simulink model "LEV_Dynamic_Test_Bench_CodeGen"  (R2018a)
settings: Solver=VariableStepAuto  StartTime=0  StopTime=37  RelTol=1e-3
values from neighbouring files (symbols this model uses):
  Anglog_Input_Max = 10    [Panda_BEVintage_VPE_S_Data_CodeGen_Model.m]    (also in ParameterInitializationFileFinal.m = 3; Panda_BEVintage_VPE_S_Data_Enhanced_Model.m)
  Anglog_Input_Min = -10    [Panda_BEVintage_VPE_S_Data_CodeGen_Model.m]    (also in ParameterInitializationFileFinal.m = 0; Panda_BEVintage_VPE_S_Data_Enhanced_Model.m)
  Anglog_Output_Max = 10    [Panda_BEVintage_VPE_S_Data_CodeGen_Model.m]    (also in Panda_BEVintage_VPE_S_Data_Enhanced_Model.m)
  Anglog_Output_Min = -10    [Panda_BEVintage_VPE_S_Data_CodeGen_Model.m]    (also in Panda_BEVintage_VPE_S_Data_Enhanced_Model.m)
  Bits = 16    [Panda_BEVintage_VPE_S_Data_CodeGen_Model.m]    (also in ParameterInitializationFileFinal.m = 12; Panda_BEVintage_VPE_S_Data_Enhanced_Model.m)
  c_1 = 0    [Panda_BEVintage_VPE_S_Data_CodeGen_Model.m]    (also in Panda_BEVintage_VPE_S_Data_Enhanced_Model.m)
  Full_BTrq_Range = Max_BTrq-Min_BTrq    (= 132)    [Panda_BEVintage_VPE_S_Data_CodeGen_Model.m]    (also in Panda_BEVintage_VPE_S_Data_Enhanced_Model.m)
  Full_Scale_Reading = Anglog_Input_Max-Anglog_Input_Min    (= 20)    [Panda_BEVintage_VPE_S_Data_CodeGen_Model.m]    (also in ParameterInitializationFileFinal.m = 3; Panda_BEVintage_VPE_S_Data_Enhanced_Model.m)
  Full_Speed_Range = Max_Speed-Min_Speed    (= 2513.27412287)    [Panda_BEVintage_VPE_S_Data_CodeGen_Model.m]    (also in Panda_BEVintage_VPE_S_Data_Enhanced_Model.m)
  g = 9.81    [Panda_BEVintage_VPE_S_Data_CodeGen_Model.m]    (also in Panda_BEVintage_VPE_S_Data_Enhanced_Model.m)
  m_e = 1.0359e+03    (= 1035.9)    [Panda_BEVintage_VPE_S_Data_CodeGen_Model.m]    (also in Panda_BEVintage_VPE_S_Data_Enhanced_Model.m)
  Max_BTrq = T_m_max    (= 66)    [Panda_BEVintage_VPE_S_Data_CodeGen_Model.m]    (also in Panda_BEVintage_VPE_S_Data_Enhanced_Model.m)
  Max_Speed = 400*pi    (= 1256.63706144)    [Panda_BEVintage_VPE_S_Data_CodeGen_Model.m]    (also in Panda_BEVintage_VPE_S_Data_Enhanced_Model.m)
  MaxInputBTrq = 5    [Panda_BEVintage_VPE_S_Data_CodeGen_Model.m]    (also in Panda_BEVintage_VPE_S_Data_Enhanced_Model.m)
  MaxOutputSpeedSensor = 5    [Panda_BEVintage_VPE_S_Data_CodeGen_Model.m]    (also in Panda_BEVintage_VPE_S_Data_Enhanced_Model.m)
  Min_BTrq = -T_m_max    (= -66)    [Panda_BEVintage_VPE_S_Data_CodeGen_Model.m]    (also in Panda_BEVintage_VPE_S_Data_Enhanced_Model.m)
  Min_Speed = -400*pi    (= -1256.63706144)    [Panda_BEVintage_VPE_S_Data_CodeGen_Model.m]    (also in Panda_BEVintage_VPE_S_Data_Enhanced_Model.m)
  MinInputBTrq = -5    [Panda_BEVintage_VPE_S_Data_CodeGen_Model.m]    (also in Panda_BEVintage_VPE_S_Data_Enhanced_Model.m)
  MinOutputSpeedSensor = -5    [Panda_BEVintage_VPE_S_Data_CodeGen_Model.m]    (also in Panda_BEVintage_VPE_S_Data_Enhanced_Model.m)
  r_e = 0.27    [Panda_BEVintage_VPE_S_Data_CodeGen_Model.m]    (also in Panda_BEVintage_VPE_S_Data_Enhanced_Model.m)
  Sampling_Time = 0.0001    [Panda_BEVintage_VPE_S_Data_CodeGen_Model.m]    (also in ParameterInitializationFileFinal.m = 0.01; Panda_BEVintage_VPE_S_Data_Enhanced_Model.m)
  T_m_max = 66    [Panda_BEVintage_VPE_S_Data_CodeGen_Model.m]    (also in Panda_BEVintage_VPE_S_Data_Enhanced_Model.m)
  T_r = 8.67    [Panda_BEVintage_VPE_S_Data_CodeGen_Model.m]    (also in Panda_BEVintage_VPE_S_Data_Enhanced_Model.m)
  ZOH_Time = 0.0001    [Panda_BEVintage_VPE_S_Data_CodeGen_Model.m]    (also in Panda_BEVintage_VPE_S_Data_Enhanced_Model.m)
undefined symbols (not defined in the file or in its folder): DiscIntNeverNeededParam, m, s, seconds
libraries: autolibmappedmotor x2, simulink x2, autolibshared x2, autolibsharedcoupling x1

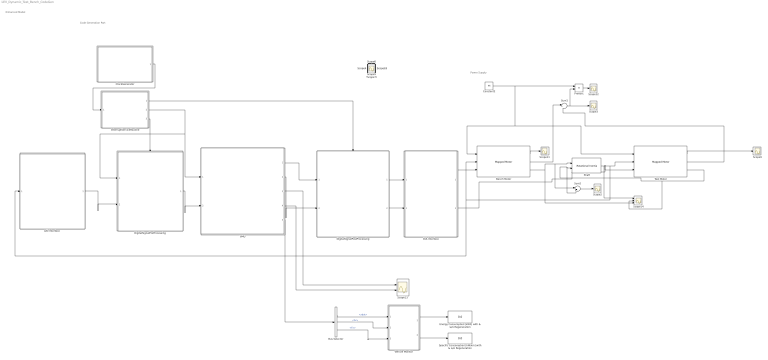
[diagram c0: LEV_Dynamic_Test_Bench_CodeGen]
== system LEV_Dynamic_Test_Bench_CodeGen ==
  note: Enhanced Model
  note: Code Generation Part
  note: Power Supply
  "A/D Interface " : Subsystem
  Bench Motor : autolibmappedmotor/Mapped Motor  port_config=Speed  param_by=Maximum torque and power  w_t=[ 0 375 750 800 ]  T_t=[0.09 0.08 0.07 0]  torque_max=T_m_max  power_max=P_m_max  Tc=tau_m  param_loss=Single efficiency measurement  eff=eta_n  w_eff=w_n  T_eff=T_m_n  Piron=Pl_iron  Pbase=Pl_eln  w_eff_bp=[-8000 -4000 0 4000 8000]  T_eff_bp=[0 0.03 0.06 0.09]  losses_table=[1 2;3 4]  efficiency_table=[95 95 95 95; 95 95 95 95; 95 95 95 95; 95 95 95 95; 95 95 95 95]  J=5e-6  b=1e-5  omega_o=0  T_t_extended=[0 0.07 0.08 0.09 0.08 0.07 0]  w_t_extended=[-800 -750 -375 0 375 750 800]  KLossIron=0  KLossCopper=0.68708  x_w_eff_vec=[-400 0 400]  x_T_eff_vec=[-20 0 20]  x_losses_mat=[4 3 4;2 1 2;4 3 4]  aMode=aMode
  Bus Selector : BusSelector  OutputSignals=BdyFrm.Cg.Vel.xdot,BdyFrm.Forces.Ext.Fx,BdyFrm.Forces.Drag.Fx
  ClockGenerator : Subsystem
  Constant2 : Constant  Value=96
  D/A Interface : Subsystem
  DigitalSignalPostProcessing : Subsystem
  DigitalSignalPreProcessing : Subsystem
  Energy Consumption [kWh] with & w/o Regeneration : Display
  InterruptServiceRoutine : Subsystem
  Product : Product
  Scope{,1..12,18} (14 alike) : Scope
  Scope13 : Scope  NumInputPorts=2
  Scope14 : Scope  NumInputPorts=3
  Shaft : autolibsharedcoupling/Rotational Inertia  port_config=Simulink  J=.01  b=.001  omega_o=0  externJ=off  blkID=0  aMode=1
  Specific Consumption [kW/km] with & w/o Regeneration : Display
  Sum1 : Sum  Inputs=|++
  Sum2 : Sum  Inputs=|++
  Test Motor : autolibmappedmotor/Mapped Motor  port_config=Speed  param_by=Maximum torque and power  w_t=[ 0 375 750 800 ]  T_t=[0.09 0.08 0.07 0]  torque_max=T_m_max  power_max=P_m_max  Tc=tau_m  param_loss=Single efficiency measurement  eff=eta_n  w_eff=w_n  T_eff=T_m_n  Piron=Pl_iron  Pbase=Pl_eln  w_eff_bp=[-8000 -4000 0 4000 8000]  T_eff_bp=[0 0.03 0.06 0.09]  losses_table=[1 2;3 4]  efficiency_table=[95 95 95 95; 95 95 95 95; 95 95 95 95; 95 95 95 95; 95 95 95 95]  J=5e-6  b=1e-5  omega_o=0  T_t_extended=[0 0.07 0.08 0.09 0.08 0.07 0]  w_t_extended=[-800 -750 -375 0 375 750 800]  KLossIron=0  KLossCopper=0.68708  x_w_eff_vec=[-400 0 400]  x_T_eff_vec=[-20 0 20]  x_losses_mat=[4 3 4;2 1 2;4 3 4]  aMode=aMode
  VMU : Subsystem
  Vehicle Monitor : Subsystem
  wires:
  Test Motor/3 -> Scope14/2, Shaft/2, Sum2/2
  Bench Motor/3 -> Scope14/3, Sum2/1, Shaft/1
  Constant2/1 -> Bench Motor/1, Test Motor/1, Product/1
  Shaft/1 -> Scope14/1, "A/D Interface "/1(ShaftSpeed), Bench Motor/2, Test Motor/2
  Test Motor/2 -> Sum1/2
  Sum1/1 -> Product/2, Scope3/1
  Bench Motor/2 -> Sum1/1
  Sum2/1 -> Scope2/1
  Bench Motor/1 -> Scope11/1
  Test Motor/1 -> Scope9/1
  Product/1 -> Scope12/1
  Bus Selector/1 -> Vehicle Monitor/1(In1)  "<xdot>"
  Bus Selector/3 -> Vehicle Monitor/3(In3)  "<Fx>"
  Bus Selector/2 -> Vehicle Monitor/2(In2)  "<Fx>"
  Vehicle Monitor/1(Out1) -> Energy Consumption [kWh] with & w/o Regeneration/1
  Vehicle Monitor/2(Out2) -> Specific Consumption [kW/km] with & w/o Regeneration/1
  D/A Interface/1("BenchTrqCMD ") -> Bench Motor/3
  D/A Interface/2("MotorTrqCMD ") -> Test Motor/3
  VMU/3(Speed [m/s]) -> Scope13/1
  VMU/4(ForceTot) -> Scope13/2
  VMU/5(VehicleBodyInfo) -> Bus Selector/1
  "A/D Interface "/1(ShaftSpeedDigitalSignal) -> DigitalSignalPreProcessing/2(ShaftSpeedDigitalSignal)
  DigitalSignalPreProcessing/1("AverageShaftSpeedDigitalSignal ") -> VMU/2("AverageShaftSpeedDigitalSignal ")
  ClockGenerator/1(ClkSignal) -> InterruptServiceRoutine/1(ClkSignal)
  DigitalSignalPostProcessing/1(BenchTrqCMD16Bits) -> D/A Interface/1(DigitalBenchTrqCMD)
  DigitalSignalPostProcessing/2(MotorTrqCMD16Bits) -> D/A Interface/2(DigitalMotorTrqCMD)
  VMU/2(MotorTrqCMD) -> DigitalSignalPostProcessing/2(MotorTrqCMD)
  VMU/1(BenchTrqCMD) -> DigitalSignalPostProcessing/1(BenchTrqCMD)
  InterruptServiceRoutine/2(CoreTrigger) -> VMU/1(ClkVMU), DigitalSignalPreProcessing/1(PeriodicAvgExtraction)
  InterruptServiceRoutine/3(PreTrigger) -> DigitalSignalPreProcessing/Trigger
  InterruptServiceRoutine/1(PostEnable) -> DigitalSignalPostProcessing/Enable

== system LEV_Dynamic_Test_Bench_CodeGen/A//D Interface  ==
  ShaftSpeed : Inport
  ADC BOUNDARY : Subsystem
  LinearTransducer : Subsystem
  Signal Scaling to Adapt Target Input Dynamics : Subsystem
  ShaftSpeedDigitalSignal : Outport
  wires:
  Signal Scaling to Adapt Target Input Dynamics/1(SignalScaledToTargetDynamics -10 to +10 [V]) -> ADC BOUNDARY/1(ShaftSpeedSignal)
  ADC BOUNDARY/1(ShaftSpeedDigitalSignal) -> ShaftSpeedDigitalSignal/1
  ShaftSpeed/1 -> LinearTransducer/1("ShaftSpeed ")
  LinearTransducer/1(SpeedSensorOutputVoltage -5 to +5 [V]) -> Signal Scaling to Adapt Target Input Dynamics/1("SpeedSensorOutputVoltage ")

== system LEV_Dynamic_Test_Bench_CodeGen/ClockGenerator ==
  MainClk : DiscretePulseGenerator  PulseType=Time based  Period=Sampling_Time/10
  ClkSignal : Outport
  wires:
  MainClk/1 -> ClkSignal/1

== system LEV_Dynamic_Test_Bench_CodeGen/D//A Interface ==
  DigitalBenchTrqCMD : Inport
  DigitalMotorTrqCMD : Inport  Port=2
  DAC BOUNDARY : Subsystem
  LinearActuator : Subsystem
  Signal Scaling to Bench Dynamics : Subsystem
  "BenchTrqCMD " : Outport
  "MotorTrqCMD " : Outport  Port=2
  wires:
  DAC BOUNDARY/1(AnalogBenchTrqCMD -10 to +10 V) -> Signal Scaling to Bench Dynamics/1(" AnalogBenchTrqCMD -10 to +10 V ")
  DAC BOUNDARY/2("AnalogMotorTrqCMD -10 to +10 V ") -> Signal Scaling to Bench Dynamics/2("AnalogMotorTrqCMD -10 to +10 V ")
  LinearActuator/1(BenchTrqCMD) -> "BenchTrqCMD "/1
  Signal Scaling to Bench Dynamics/1(BenchTrqCmdInVolts) -> LinearActuator/1(BenchTrqCmdInVolts)
  Signal Scaling to Bench Dynamics/2(MotorTrqCmdInVolts) -> LinearActuator/2(MotorTrqCmdInVolts)
  LinearActuator/2(MotorTrqCMD) -> "MotorTrqCMD "/1
  DigitalBenchTrqCMD/1 -> DAC BOUNDARY/1(BenchTrqCMD16Bits)
  DigitalMotorTrqCMD/1 -> DAC BOUNDARY/2(MotorTrqCMD16Bits)

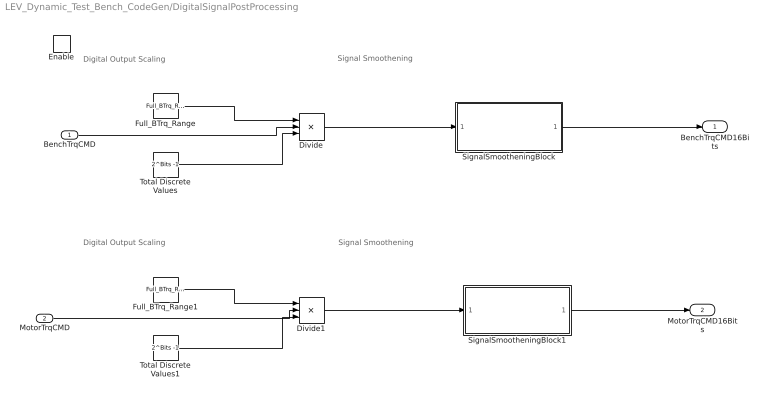
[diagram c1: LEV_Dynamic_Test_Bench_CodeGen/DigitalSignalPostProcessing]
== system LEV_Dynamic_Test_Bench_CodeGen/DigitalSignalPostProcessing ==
  note: Digital Output Scaling
  note: Digital Output Scaling
  note: Signal Smoothening
  note: Signal Smoothening
  BenchTrqCMD : Inport
  MotorTrqCMD : Inport  Port=2
  Enable : EnablePort
  Divide : Product  Inputs=/**
  Divide1 : Product  Inputs=/**
  Full_BTrq_Range : Constant  Value=Full_BTrq_Range
  Full_BTrq_Range1 : Constant  Value=Full_BTrq_Range
  SignalSmootheningBlock : Subsystem
  SignalSmootheningBlock1 : Subsystem
  Total Discrete Values : Constant  Value=2^Bits -1
  Total Discrete Values1 : Constant  Value=2^Bits -1
  BenchTrqCMD16Bits : Outport
  MotorTrqCMD16Bits : Outport  Port=2
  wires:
  BenchTrqCMD/1 -> Divide/2
  Full_BTrq_Range/1 -> Divide/1
  Total Discrete Values/1 -> Divide/3
  Total Discrete Values1/1 -> Divide1/3
  MotorTrqCMD/1 -> Divide1/2
  Full_BTrq_Range1/1 -> Divide1/1
  Divide1/1 -> SignalSmootheningBlock1/1(SignalIn)
  Divide/1 -> SignalSmootheningBlock/1(SignalIn)
  SignalSmootheningBlock/1(SmoothSignal) -> BenchTrqCMD16Bits/1
  SignalSmootheningBlock1/1(SmoothSignal) -> MotorTrqCMD16Bits/1

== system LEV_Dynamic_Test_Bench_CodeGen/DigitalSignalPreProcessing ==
  PeriodicAvgExtraction : Inport
  ShaftSpeedDigitalSignal : Inport  Port=2
  Trigger : TriggerPort  VariantControl=Variant  PortDimensions=1
  DigitalSignalScaling : Subsystem
  Signal Averaging Block : Subsystem
  "AverageShaftSpeedDigitalSignal " : Outport
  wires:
  DigitalSignalScaling/1("ShaftSpeedDigitalSignal ") -> Signal Averaging Block/1("ShaftSpeedDigitalSignal ")
  Signal Averaging Block/1("AverageShaftSpeedDigitalSignal ") -> "AverageShaftSpeedDigitalSignal "/1
  PeriodicAvgExtraction/1 -> Signal Averaging Block/2(PeriodicAvgExtraction)
  ShaftSpeedDigitalSignal/1 -> DigitalSignalScaling/1(ShaftSpeedDigitalSignal)

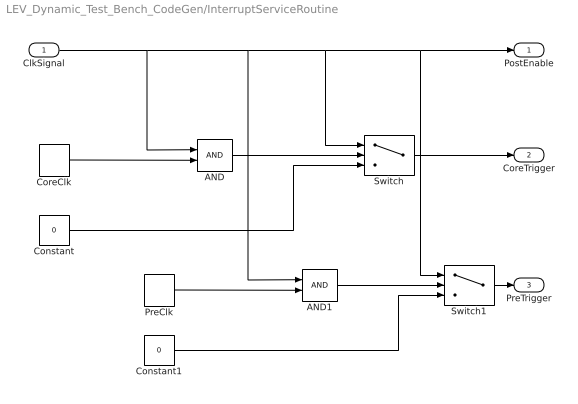
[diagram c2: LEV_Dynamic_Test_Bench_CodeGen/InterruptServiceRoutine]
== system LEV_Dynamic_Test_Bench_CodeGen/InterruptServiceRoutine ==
  ClkSignal : Inport
  AND : Logic  IconShape=distinctive  AllPortsSameDT=off  OutDataTypeStr=boolean
  AND1 : Logic  IconShape=distinctive  AllPortsSameDT=off  OutDataTypeStr=boolean
  Constant : Constant  Value=0
  Constant1 : Constant  Value=0
  CoreClk : DiscretePulseGenerator  PulseType=Time based  Period=Sampling_Time*10
  PreClk : DiscretePulseGenerator  PulseType=Time based  Period=Sampling_Time
  Switch : Switch  Criteria=u2 > Threshold
  Switch1 : Switch  Criteria=u2 > Threshold
  PostEnable : Outport
  CoreTrigger : Outport  Port=2
  PreTrigger : Outport  Port=3
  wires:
  Switch/1 -> CoreTrigger/1
  AND/1 -> Switch/2
  Constant/1 -> Switch/3
  CoreClk/1 -> AND/2
  PreClk/1 -> AND1/2
  ClkSignal/1 -> AND/1, AND1/1, Switch/1, Switch1/1, PostEnable/1
  AND1/1 -> Switch1/2
  Constant1/1 -> Switch1/3
  Switch1/1 -> PreTrigger/1

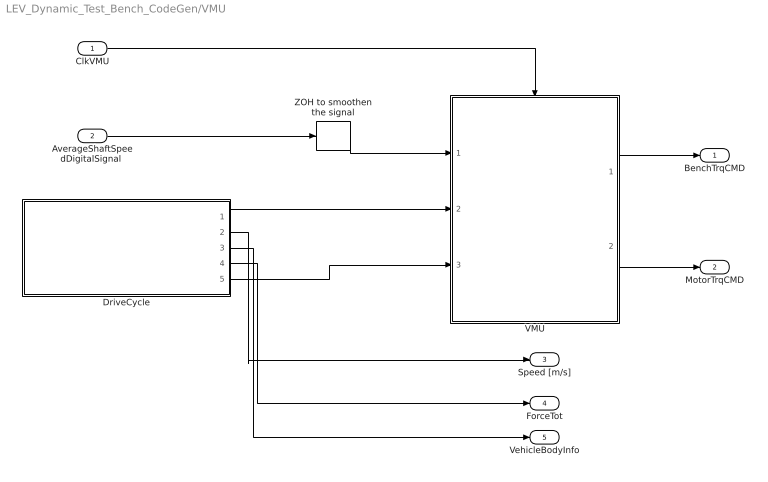
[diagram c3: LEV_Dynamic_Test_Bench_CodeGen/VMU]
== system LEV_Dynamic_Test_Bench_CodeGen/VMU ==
  ClkVMU : Inport
  "AverageShaftSpeedDigitalSignal " : Inport  Port=2
  DriveCycle : Subsystem
  VMU : Subsystem
  ZOH to smoothen the signal : ZeroOrderHold  SampleTime=Sampling_Time*10
  BenchTrqCMD : Outport
  MotorTrqCMD : Outport  Port=2
  Speed [m/s] : Outport  Port=3
  ForceTot : Outport  Port=4
  VehicleBodyInfo : Outport  Port=5
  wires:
  DriveCycle/2(Speed) -> Speed [m/s]/1
  DriveCycle/3(VehicleBodyInfo) -> VehicleBodyInfo/1
  DriveCycle/4(ForceTotal) -> ForceTot/1
  DriveCycle/1(ShaftSpeed) -> VMU/2(ShaftSpeed)
  DriveCycle/5(MotorTrqCMD) -> VMU/3(MotorTrq)
  VMU/1(BenchTrqCMD) -> BenchTrqCMD/1
  VMU/2(MotorTrqCMD) -> MotorTrqCMD/1
  "AverageShaftSpeedDigitalSignal "/1 -> ZOH to smoothen the signal/1
  ZOH to smoothen the signal/1 -> VMU/1(AvgShaftSpeedFedBack)
  ClkVMU/1 -> VMU/Trigger

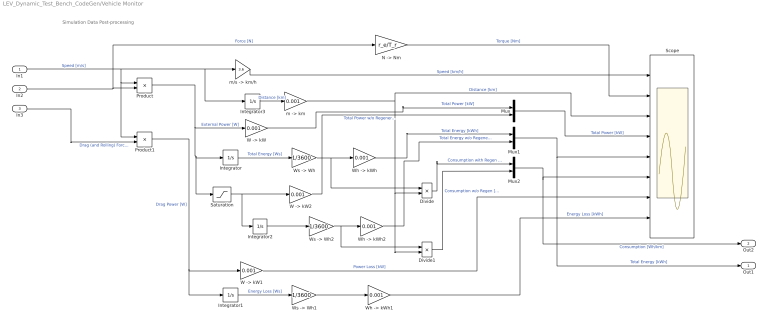
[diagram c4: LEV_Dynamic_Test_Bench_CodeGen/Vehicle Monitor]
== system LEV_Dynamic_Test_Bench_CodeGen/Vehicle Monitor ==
  note: Simulation Data Post-processing
  In1 : Inport
  In2 : Inport  Port=2
  In3 : Inport  Port=3
  Divide : Product  Inputs=*/
  Divide1 : Product  Inputs=*/
  Integrator{,1..3} (4 alike) : Integrator
  Mux : Mux  Inputs=2
  Mux1 : Mux  Inputs=2
  Mux2 : Mux  Inputs=2
  "N -> Nm" : Gain  Gain=r_e/T_r
  Product : Product
  Product1 : Product
  Saturation : Saturate  UpperLimit=inf  LowerLimit=0
  Scope : Scope  NumInputPorts=8
  "W -> kW" : Gain  Gain=0.001
  "W -> kW1" : Gain  Gain=0.001
  "W -> kW2" : Gain  Gain=0.001
  "Wh -> kWh" : Gain  Gain=0.001
  "Wh -> kWh1" : Gain  Gain=0.001
  "Wh -> kWh2" : Gain  Gain=0.001
  "Ws -> Wh" : Gain  Gain=1/3600
  "Ws -> Wh1" : Gain  Gain=1/3600
  "Ws -> Wh2" : Gain  Gain=1/3600
  "m -> km" : Gain  Gain=0.001
  "m/s -> km/h" : Gain  Gain=3.6
  Out1 : Outport
  Out2 : Outport  Port=2
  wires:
  Divide/1 -> Mux2/1  "Consumption with Regen [Wh/km]"
  "Wh -> kWh1"/1 -> Scope/8  "Energy Loss [kWh]"
  Saturation/1 -> Integrator2/1, "W -> kW2"/1
  "Wh -> kWh2"/1 -> Mux1/2  "Total Energy w/o Regeneration [kWh]"
  Mux1/1 -> Out1/1, Scope/5  "Total Energy [kWh]"
  "W -> kW"/1 -> Mux/1  "Total Power [kW]"
  Divide1/1 -> Mux2/2  "Consumption w/o Regen [Wh/km]"
  "Wh -> kWh"/1 -> Mux1/1  "Total Energy [kWh]"
  "W -> kW1"/1 -> Scope/7  "Power Loss [kW]"
  Integrator/1 -> "Ws -> Wh"/1  "Total Energy [Ws]"
  Integrator1/1 -> "Ws -> Wh1"/1  "Energy Loss [Ws]"
  "Ws -> Wh2"/1 -> Divide1/1, "Wh -> kWh2"/1
  Product1/1 -> Integrator1/1, "W -> kW1"/1  "Drag Power [W]"
  "N -> Nm"/1 -> Scope/2  "Torque [Nm]"
  Mux/1 -> Scope/4  "Total Power [kW]"
  "W -> kW2"/1 -> Mux/2  "Total Power w/o Regeneration [kW]"
  Mux2/1 -> Out2/1, Scope/6  "Consumption [Wh/km]"
  Integrator2/1 -> "Ws -> Wh2"/1
  "Ws -> Wh1"/1 -> "Wh -> kWh1"/1
  "m -> km"/1 -> Scope/3, Divide1/2, Divide/2  "Distance [km]"
  In2/1 -> "N -> Nm"/1, Product/2  "Force [N]"
  Product/1 -> Saturation/1, Integrator/1, "W -> kW"/1  "External Power [W]"
  "Ws -> Wh"/1 -> Divide/1, "Wh -> kWh"/1
  Integrator3/1 -> "m -> km"/1  "Distance [km]"
  "m/s -> km/h"/1 -> Scope/1  "Speed [km/h]"
  In1/1 -> Product1/1, Product/1, "m/s -> km/h"/1, Integrator3/1  "Speed [m/s]"
  In3/1 -> Product1/2  "Drag (and Rolling) Force [N]"

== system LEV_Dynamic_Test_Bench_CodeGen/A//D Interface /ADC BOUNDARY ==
  note: Quantizer
  note: Time Sampling Block
  note: Digital Output
  note: Clamped Signal
  note: ADC
  ShaftSpeedSignal : Inport
  Divide : Product  Inputs=/**
  Full_Scale_Reading : Constant  Value=Full_Scale_Reading
  Quantizer : Quantizer  QuantizationInterval=Full_Scale_Reading/(2^Bits-1 )
  Signal Clamper : Saturate  UpperLimit=Anglog_Input_Max  LowerLimit=Anglog_Input_Min
  Total Discrete Values : Constant  Value=2^Bits -1
  Zero-Order Hold2 : ZeroOrderHold  SampleTime=Sampling_Time
  ShaftSpeedDigitalSignal : Outport
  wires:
  Signal Clamper/1 -> Zero-Order Hold2/1
  ShaftSpeedSignal/1 -> Signal Clamper/1
  Full_Scale_Reading/1 -> Divide/1
  Total Discrete Values/1 -> Divide/3
  Quantizer/1 -> Divide/2  "uspq(z)"
  Divide/1 -> ShaftSpeedDigitalSignal/1  "Digital Signal ud(z)"
  Zero-Order Hold2/1 -> Quantizer/1  "usp(z)"

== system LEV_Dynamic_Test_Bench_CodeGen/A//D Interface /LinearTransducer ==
  "ShaftSpeed " : Inport
  Add : Sum
  Offset Term c : Subsystem
  Product : Product
  Scaling Coefficient m : Subsystem
  Signal Specification : SignalSpecification  Unit=V
  SpeedSensorOutputVoltage -5 to +5 [V] : Outport
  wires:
  Add/1 -> Signal Specification/1
  Scaling Coefficient m/1(Scaling Coefficient m) -> Product/1, Offset Term c/1(Scaling Coefficent m)
  Product/1 -> Add/2
  Offset Term c/1("Offset Term c ") -> Add/1
  "ShaftSpeed "/1 -> Product/2
  Signal Specification/1 -> SpeedSensorOutputVoltage -5 to +5 [V]/1

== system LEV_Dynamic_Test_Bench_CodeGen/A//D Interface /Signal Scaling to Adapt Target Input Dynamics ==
  "SpeedSensorOutputVoltage " : Inport
  Add : Sum
  Offset Term c : Subsystem
  Product : Product
  Scaling Coefficient m : Subsystem
  Signal Specification : SignalSpecification  Unit=V
  SignalScaledToTargetDynamics -10 to +10 [V] : Outport
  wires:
  Scaling Coefficient m/1(Scaling Coefficient m) -> Product/1, Offset Term c/1(Scaling Coefficent m)
  "SpeedSensorOutputVoltage "/1 -> Product/2
  Product/1 -> Add/2
  Offset Term c/1("Offset Term c ") -> Add/1
  Add/1 -> Signal Specification/1
  Signal Specification/1 -> SignalScaledToTargetDynamics -10 to +10 [V]/1

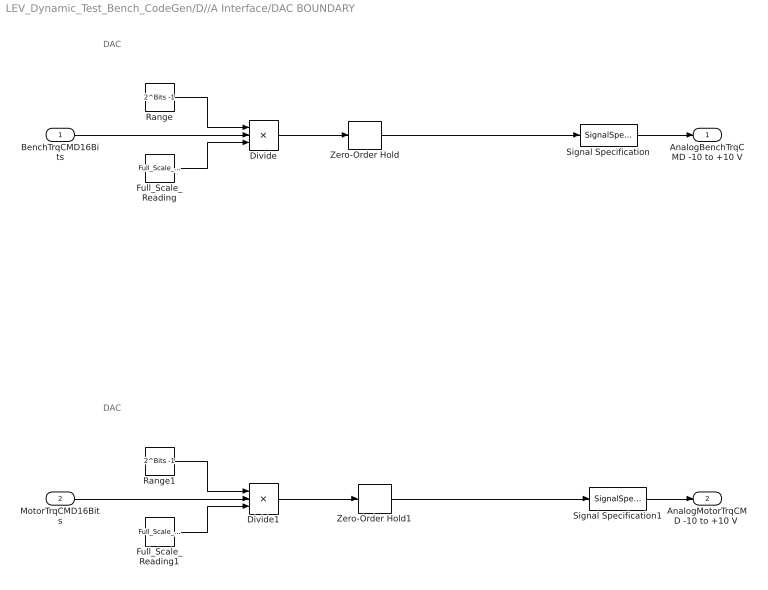
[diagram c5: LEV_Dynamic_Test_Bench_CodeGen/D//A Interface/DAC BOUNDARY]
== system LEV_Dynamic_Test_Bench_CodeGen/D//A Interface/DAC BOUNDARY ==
  note: DAC
  note: DAC
  BenchTrqCMD16Bits : Inport
  MotorTrqCMD16Bits : Inport  Port=2
  Divide : Product  Inputs=/**
  Divide1 : Product  Inputs=/**
  Full_Scale_Reading : Constant  Value=Full_Scale_Reading
  Full_Scale_Reading1 : Constant  Value=Full_Scale_Reading
  Range : Constant  Value=2^Bits -1
  Range1 : Constant  Value=2^Bits -1
  Signal Specification : SignalSpecification  Unit=V
  Signal Specification1 : SignalSpecification  Unit=V
  Zero-Order Hold : ZeroOrderHold  SampleTime=ZOH_Time
  Zero-Order Hold1 : ZeroOrderHold  SampleTime=ZOH_Time
  AnalogBenchTrqCMD -10 to +10 V : Outport
  "AnalogMotorTrqCMD -10 to +10 V " : Outport  Port=2
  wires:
  Range/1 -> Divide/1
  Full_Scale_Reading/1 -> Divide/3
  BenchTrqCMD16Bits/1 -> Divide/2
  Divide/1 -> Zero-Order Hold/1
  Full_Scale_Reading1/1 -> Divide1/3
  Divide1/1 -> Zero-Order Hold1/1
  MotorTrqCMD16Bits/1 -> Divide1/2
  Range1/1 -> Divide1/1
  Signal Specification1/1 -> "AnalogMotorTrqCMD -10 to +10 V "/1
  Signal Specification/1 -> AnalogBenchTrqCMD -10 to +10 V/1
  Zero-Order Hold1/1 -> Signal Specification1/1
  Zero-Order Hold/1 -> Signal Specification/1

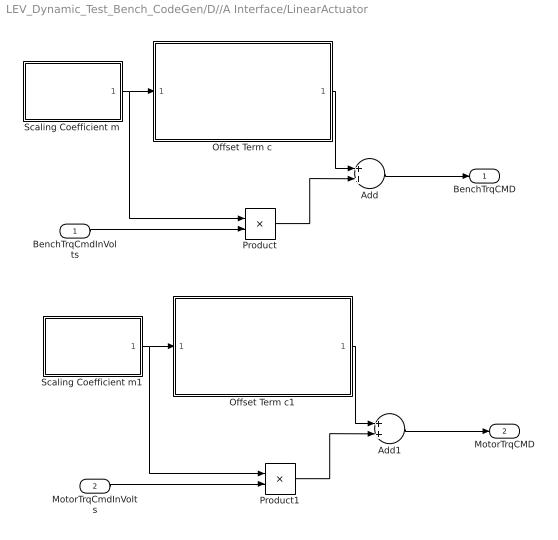
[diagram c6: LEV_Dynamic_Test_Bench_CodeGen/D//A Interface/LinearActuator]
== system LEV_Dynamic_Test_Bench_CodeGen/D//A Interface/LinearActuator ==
  BenchTrqCmdInVolts : Inport
  MotorTrqCmdInVolts : Inport  Port=2
  Add : Sum
  Add1 : Sum
  Offset Term c : Subsystem
  Offset Term c1 : Subsystem
  Product : Product
  Product1 : Product
  Scaling Coefficient m : Subsystem
  Scaling Coefficient m1 : Subsystem
  BenchTrqCMD : Outport
  MotorTrqCMD : Outport  Port=2
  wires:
  Add/1 -> BenchTrqCMD/1
  Scaling Coefficient m/1(Scaling Coefficient m) -> Product/1, Offset Term c/1(Scaling Coefficent m)
  Product/1 -> Add/2
  Offset Term c/1("Offset Term c ") -> Add/1
  BenchTrqCmdInVolts/1 -> Product/2
  MotorTrqCmdInVolts/1 -> Product1/2
  Scaling Coefficient m1/1(Scaling Coefficient m) -> Product1/1, Offset Term c1/1(Scaling Coefficent m)
  Product1/1 -> Add1/2
  Add1/1 -> MotorTrqCMD/1
  Offset Term c1/1("Offset Term c ") -> Add1/1

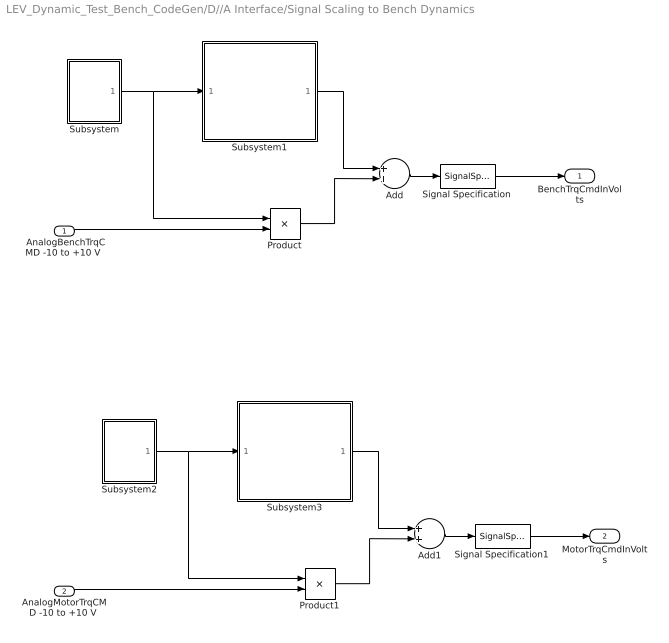
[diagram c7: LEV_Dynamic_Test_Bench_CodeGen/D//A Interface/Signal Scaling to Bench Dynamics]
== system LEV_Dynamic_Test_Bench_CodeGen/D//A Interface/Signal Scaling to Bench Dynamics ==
  " AnalogBenchTrqCMD -10 to +10 V " : Inport
  "AnalogMotorTrqCMD -10 to +10 V " : Inport  Port=2
  Add : Sum
  Add1 : Sum
  Product : Product
  Product1 : Product
  Signal Specification : SignalSpecification  Unit=V
  Signal Specification1 : SignalSpecification  Unit=V
  Subsystem : Subsystem
  Subsystem1 : Subsystem
  Subsystem2 : Subsystem
  Subsystem3 : Subsystem
  BenchTrqCmdInVolts : Outport
  MotorTrqCmdInVolts : Outport  Port=2
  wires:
  Product/1 -> Add/2
  Add/1 -> Signal Specification/1
  Subsystem/1("Gradient ") -> Product/1, Subsystem1/1("Gradient ")
  Subsystem1/1("Offset ") -> Add/1
  " AnalogBenchTrqCMD -10 to +10 V "/1 -> Product/2
  Add1/1 -> Signal Specification1/1
  "AnalogMotorTrqCMD -10 to +10 V "/1 -> Product1/2
  Subsystem3/1("Offset ") -> Add1/1
  Subsystem2/1("Gradient ") -> Product1/1, Subsystem3/1("Gradient ")
  Product1/1 -> Add1/2
  Signal Specification1/1 -> MotorTrqCmdInVolts/1
  Signal Specification/1 -> BenchTrqCmdInVolts/1

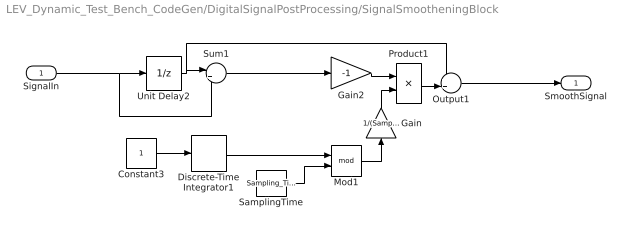
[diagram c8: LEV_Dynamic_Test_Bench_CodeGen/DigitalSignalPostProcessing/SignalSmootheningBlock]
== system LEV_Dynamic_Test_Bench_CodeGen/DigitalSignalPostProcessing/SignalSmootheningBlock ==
  SignalIn : Inport
  Constant3 : Constant
  Discrete-Time Integrator1 : DiscreteIntegrator  SampleTime=Sampling_Time/10  ICPrevOutput=DiscIntNeverNeededParam  ICPrevScaledInput=DiscIntNeverNeededParam
  Gain : Gain  Gain=1/(Sampling_Time*10)
  Gain2 : Gain  DisableCoverage=on  Gain=-1
  Mod1 : Math  Operator=mod
  Output1 : Sum  Inputs=++|
  Product1 : Product  DisableCoverage=on
  SamplingTime : Constant  Value=Sampling_Time*10
  Sum1 : Sum  DisableCoverage=on  Inputs=|+-
  Unit Delay2 : UnitDelay  SampleTime=Sampling_Time*10
  SmoothSignal : Outport
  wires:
  Sum1/1 -> Gain2/1
  Unit Delay2/1 -> Output1/1, Sum1/1
  Gain2/1 -> Product1/1
  Output1/1 -> SmoothSignal/1
  Product1/1 -> Output1/2
  SignalIn/1 -> Sum1/2, Unit Delay2/1
  SamplingTime/1 -> Mod1/2
  Discrete-Time Integrator1/1 -> Mod1/1
  Constant3/1 -> Discrete-Time Integrator1/1
  Mod1/1 -> Gain/1
  Gain/1 -> Product1/2

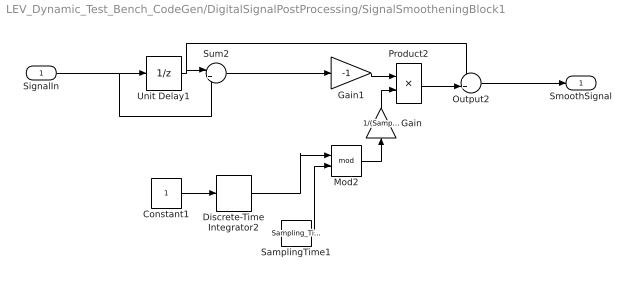
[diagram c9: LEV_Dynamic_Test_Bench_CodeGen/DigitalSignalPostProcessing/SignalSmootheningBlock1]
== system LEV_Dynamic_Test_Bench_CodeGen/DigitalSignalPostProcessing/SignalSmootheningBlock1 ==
  SignalIn : Inport
  Constant1 : Constant
  Discrete-Time Integrator2 : DiscreteIntegrator  SampleTime=Sampling_Time/10  ICPrevOutput=DiscIntNeverNeededParam  ICPrevScaledInput=DiscIntNeverNeededParam
  Gain : Gain  Gain=1/(Sampling_Time*10)
  Gain1 : Gain  DisableCoverage=on  Gain=-1
  Mod2 : Math  Operator=mod
  Output2 : Sum  Inputs=++|
  Product2 : Product  DisableCoverage=on
  SamplingTime1 : Constant  Value=Sampling_Time*10
  Sum2 : Sum  DisableCoverage=on  Inputs=|+-
  Unit Delay1 : UnitDelay  SampleTime=Sampling_Time*10
  SmoothSignal : Outport
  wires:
  Gain/1 -> Product2/2
  Constant1/1 -> Discrete-Time Integrator2/1
  Discrete-Time Integrator2/1 -> Mod2/1
  SamplingTime1/1 -> Mod2/2
  Sum2/1 -> Gain1/1
  SignalIn/1 -> Sum2/2, Unit Delay1/1
  Output2/1 -> SmoothSignal/1
  Gain1/1 -> Product2/1
  Unit Delay1/1 -> Output2/1, Sum2/1
  Mod2/1 -> Gain/1
  Product2/1 -> Output2/2

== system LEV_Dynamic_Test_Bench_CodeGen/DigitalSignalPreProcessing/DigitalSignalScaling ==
  ShaftSpeedDigitalSignal : Inport
  ScalingToSignalValues : Subsystem
  "ShaftSpeedDigitalSignal " : Outport
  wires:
  ShaftSpeedDigitalSignal/1 -> ScalingToSignalValues/1(ShaftSpeedDigitalSignal)
  ScalingToSignalValues/1("ShaftSpeedDigitalSignal ") -> "ShaftSpeedDigitalSignal "/1

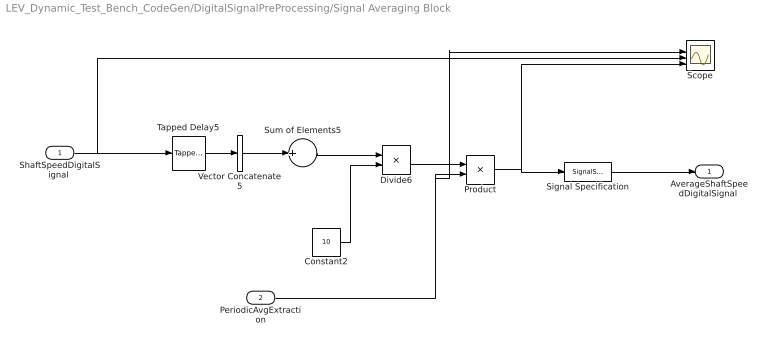
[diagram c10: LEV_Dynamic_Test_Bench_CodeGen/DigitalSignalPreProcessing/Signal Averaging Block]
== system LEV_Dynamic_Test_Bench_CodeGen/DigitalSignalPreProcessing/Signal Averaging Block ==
  "ShaftSpeedDigitalSignal " : Inport
  PeriodicAvgExtraction : Inport  Port=2
  Constant2 : Constant  Value=10
  Divide6 : Product  Inputs=*/
  Product : Product
  Scope : Scope  NumInputPorts=4
  Signal Specification : SignalSpecification  Unit=rad/s
  Sum of Elements5 : Sum  Inputs=+
  Tapped Delay5 : simulink/Discrete/Tapped Delay  vinit=0.0  samptime=-1  NumDelays=10  DelayOrder=Oldest  includeCurrent=off
  Vector Concatenate5 : Concatenate  NumInputs=1
  "AverageShaftSpeedDigitalSignal " : Outport
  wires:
  Vector Concatenate5/1 -> Sum of Elements5/1
  Sum of Elements5/1 -> Divide6/1
  Constant2/1 -> Divide6/2
  "ShaftSpeedDigitalSignal "/1 -> Scope/3, Tapped Delay5/1
  Tapped Delay5/1 -> Vector Concatenate5/1
  Divide6/1 -> Product/1
  PeriodicAvgExtraction/1 -> Scope/2, Product/2
  Product/1 -> Scope/4, Signal Specification/1
  Signal Specification/1 -> "AverageShaftSpeedDigitalSignal "/1

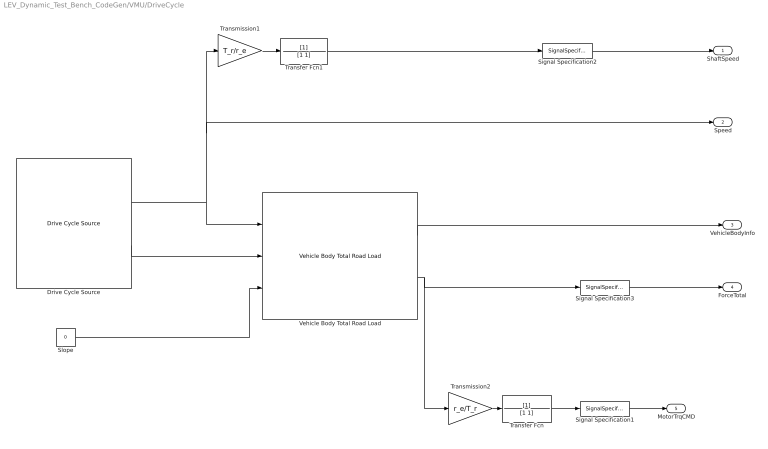
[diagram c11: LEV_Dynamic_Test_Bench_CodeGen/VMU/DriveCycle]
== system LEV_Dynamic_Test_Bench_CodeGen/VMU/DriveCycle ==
  Drive Cycle Source : autolibshared/Drive Cycle Source  cycleVar=FTP75  fileVar=cycleFTP75.mat  tfinal="2474  seconds"  cycleRepeat=off  outAccPort=on  outGearPort=off  gearList=No gear data  t_wot1=5  xdot_woto=0  xdot_wot1=10  t_wot2=20  xdot_wot2=0  t_wotend=30  srcUnit=m/s  outUnit=m/s  srcAccUnit=m/s/s  outAccUnit=m/s^2  dt=0  aMode=aMode
  Signal Specification1 : SignalSpecification  Unit=N*m
  Signal Specification2 : SignalSpecification  Unit=rad/s
  Signal Specification3 : SignalSpecification  Unit=N
  Slope : Constant  Value=0
  Transfer Fcn : TransferFcn  Denominator=[1 1]
  Transfer Fcn1 : TransferFcn  Denominator=[1 1]
  Transmission1 : Gain  Gain=T_r/r_e
  Transmission2 : Gain  Gain=r_e/T_r
  Vehicle Body Total Road Load : autolibshared/Vehicle Body Total Road Load  VariantControl=SL1dof  input_type=Kinematic  aMode=aMode  m=m_e  a=c_0  b=c_1  c=c_2  g=g  xdot_o=0
  ShaftSpeed : Outport
  Speed : Outport  Port=2
  VehicleBodyInfo : Outport  Port=3
  ForceTotal : Outport  Port=4
  MotorTrqCMD : Outport  Port=5
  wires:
  Slope/1 -> Vehicle Body Total Road Load/3
  Drive Cycle Source/1 -> Vehicle Body Total Road Load/1, Speed/1, Transmission1/1
  Transfer Fcn1/1 -> Signal Specification2/1
  Signal Specification1/1 -> MotorTrqCMD/1
  Vehicle Body Total Road Load/2 -> Signal Specification3/1, Transmission2/1
  Transfer Fcn/1 -> Signal Specification1/1
  Transmission2/1 -> Transfer Fcn/1
  Drive Cycle Source/2 -> Vehicle Body Total Road Load/2
  Transmission1/1 -> Transfer Fcn1/1
  Vehicle Body Total Road Load/1 -> VehicleBodyInfo/1
  Signal Specification2/1 -> ShaftSpeed/1
  Signal Specification3/1 -> ForceTotal/1

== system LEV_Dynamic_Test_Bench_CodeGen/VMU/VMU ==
  note: Vehicle Management Unit
  AvgShaftSpeedFedBack : Inport
  ShaftSpeed : Inport  Port=2
  MotorTrq : Inport  Port=3
  Trigger : TriggerPort  VariantControl=Variant  PortDimensions=1
  Discrete PID Controller : simulink/Continuous/PID Controller  Controller=PID  TimeDomain=Discrete-time  SampleTime=-1  IntegratorMethod=Forward Euler  FilterMethod=Forward Euler  Form=Parallel  UseFilter=on  ControllerParametersSource=internal  P=0.5  I=0.5  D=0  N=100  InitialConditionSource=internal  InitialConditionForIntegrator=0  InitialConditionForFilter=0  ExternalReset=none  LimitOutput=off  UpperSaturationLimit=inf  LowerSaturationLimit=-inf  LinearizeAsGain=off  AntiWindupMode=none  Kb=1  TrackingMode=off  Kt=1  PParamMin=[]  PParamMax=[]  IParamMin=[]  IParamMax=[]  DParamMin=[]  DParamMax=[]  NParamMin=[]  NParamMax=[]  KbParamMin=[]  KbParamMax=[]  KtParamMin=[]  KtParamMax=[]  POutMin=[]  POutMax=[]  IOutMin=[]  IOutMax=[]  DOutMin=[]  DOutMax=[]  NOutMin=[]  NOutMax=[]  KbOutMin=[]  KbOutMax=[]  KtOutMin=[]  KtOutMax=[]  IntegratorOutMin=[]  IntegratorOutMax=[]  FilterOutMin=[]  FilterOutMax=[]  SumOutMin=[]  SumOutMax=[]  SumI1OutMin=[]  SumI1OutMax=[]  SumI2OutMin=[]  SumI2OutMax=[]  SumI3OutMin=[]  SumI3OutMax=[]  SumDOutMin=[]  SumDOutMax=[]  SaturationOutMin=[]  SaturationOutMax=[]  IntegratorContinuousStateAttributes=''  IntegratorStateMustResolveToSignalObject=off  IntegratorRTWStateStorageClass=Auto  FilterContinuousStateAttributes=''  FilterStateMustResolveToSignalObject=off  FilterRTWStateStorageClass=Auto  DifferentiatorICPrevScaledInput=0  DifferentiatorOutMin=[]  DifferentiatorOutMax=[]  FilterDiffOutCoefMin=[]  FilterDiffOutCoefMax=[]  SumDenOutMin=[]  SumDenOutMax=[]  SumNumOutMin=[]  SumNumOutMax=[]  ReciprocalOutMin=[]  ReciprocalOutMax=[]  DivideOutMin=[]  DivideOutMax=[]  TunerSelectOption=Transfer Function Based (PID Tuner App)
  Saturation : Saturate  UpperLimit=T_m_max  LowerLimit=-T_m_max
  Signal Specification : SignalSpecification  Unit=N*m
  Sum : Sum  Inputs=|+-
  BenchTrqCMD : Outport
  MotorTrqCMD : Outport  Port=2
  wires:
  ShaftSpeed/1 -> Sum/1
  Sum/1 -> Discrete PID Controller/1
  Discrete PID Controller/1 -> Saturation/1
  MotorTrq/1 -> MotorTrqCMD/1
  Signal Specification/1 -> BenchTrqCMD/1
  Saturation/1 -> Signal Specification/1
  AvgShaftSpeedFedBack/1 -> Sum/2

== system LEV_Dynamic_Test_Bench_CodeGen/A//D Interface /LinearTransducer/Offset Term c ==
  Scaling Coefficent m : Inport
  MinOutputSpeedSensor : Constant  Value=MinOutputSpeedSensor
  Min_Speed : Constant  Value=Min_Speed
  Product : Product
  Subtract2 : Sum  Inputs=+-
  "Offset Term c " : Outport
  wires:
  Min_Speed/1 -> Product/1
  Scaling Coefficent m/1 -> Product/2
  Product/1 -> Subtract2/2
  Subtract2/1 -> "Offset Term c "/1
  MinOutputSpeedSensor/1 -> Subtract2/1

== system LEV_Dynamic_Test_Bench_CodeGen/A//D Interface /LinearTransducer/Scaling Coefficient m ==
  Divide : Product  Inputs=*/
  MaxOutputSpeedSensor : Constant  Value=MaxOutputSpeedSensor
  Max_Speed : Constant  Value=Max_Speed
  MinOutputSpeedSensor : Constant  Value=MinOutputSpeedSensor
  Min_Speed : Constant  Value=Min_Speed
  Subtract : Sum  Inputs=+-
  Subtract1 : Sum  Inputs=+-
  Scaling Coefficient m : Outport
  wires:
  Divide/1 -> Scaling Coefficient m/1
  Subtract1/1 -> Divide/2
  Subtract/1 -> Divide/1
  MinOutputSpeedSensor/1 -> Subtract/2
  Min_Speed/1 -> Subtract1/2
  Max_Speed/1 -> Subtract1/1
  MaxOutputSpeedSensor/1 -> Subtract/1

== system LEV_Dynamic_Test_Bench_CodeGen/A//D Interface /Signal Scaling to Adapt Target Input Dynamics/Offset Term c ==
  Scaling Coefficent m : Inport
  Anglog_Input_Min : Constant  Value=Anglog_Input_Min
  MinOutputSpeedSensor : Constant  Value=MinOutputSpeedSensor
  Product : Product
  Subtract2 : Sum  Inputs=+-
  "Offset Term c " : Outport
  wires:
  MinOutputSpeedSensor/1 -> Product/1
  Scaling Coefficent m/1 -> Product/2
  Product/1 -> Subtract2/2
  Subtract2/1 -> "Offset Term c "/1
  Anglog_Input_Min/1 -> Subtract2/1

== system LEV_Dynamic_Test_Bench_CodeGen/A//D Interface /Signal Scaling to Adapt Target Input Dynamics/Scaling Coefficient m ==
  Anglog_Input_Max : Constant  Value=Anglog_Input_Max
  Anglog_Input_Min : Constant  Value=Anglog_Input_Min
  Divide : Product  Inputs=*/
  MaxOutputSpeedSensor : Constant  Value=MaxOutputSpeedSensor
  MinOutputSpeedSensor : Constant  Value=MinOutputSpeedSensor
  Subtract : Sum  Inputs=+-
  Subtract1 : Sum  Inputs=+-
  Scaling Coefficient m : Outport
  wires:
  Divide/1 -> Scaling Coefficient m/1
  Subtract1/1 -> Divide/2
  Subtract/1 -> Divide/1
  Anglog_Input_Min/1 -> Subtract/2
  MinOutputSpeedSensor/1 -> Subtract1/2
  MaxOutputSpeedSensor/1 -> Subtract1/1
  Anglog_Input_Max/1 -> Subtract/1

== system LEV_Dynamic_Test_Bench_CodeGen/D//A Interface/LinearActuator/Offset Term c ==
  Scaling Coefficent m : Inport
  MinInputBTrq : Constant  Value=MinInputBTrq
  Min_BTrq : Constant  Value=Min_BTrq
  Product : Product
  Subtract2 : Sum  Inputs=+-
  "Offset Term c " : Outport
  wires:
  MinInputBTrq/1 -> Product/1
  Scaling Coefficent m/1 -> Product/2
  Product/1 -> Subtract2/2
  Subtract2/1 -> "Offset Term c "/1
  Min_BTrq/1 -> Subtract2/1

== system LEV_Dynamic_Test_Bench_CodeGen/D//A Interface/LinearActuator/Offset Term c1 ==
  Scaling Coefficent m : Inport
  MinInputBTrq : Constant  Value=MinInputBTrq
  Min_BTrq : Constant  Value=Min_BTrq
  Product : Product
  Subtract2 : Sum  Inputs=+-
  "Offset Term c " : Outport
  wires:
  MinInputBTrq/1 -> Product/1
  Scaling Coefficent m/1 -> Product/2
  Product/1 -> Subtract2/2
  Subtract2/1 -> "Offset Term c "/1
  Min_BTrq/1 -> Subtract2/1

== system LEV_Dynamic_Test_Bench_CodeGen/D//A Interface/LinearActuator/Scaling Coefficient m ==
  Divide : Product  Inputs=*/
  MaxInputBTrq : Constant  Value=MaxInputBTrq
  Max_BTrq : Constant  Value=Max_BTrq
  MinInputBTrq : Constant  Value=MinInputBTrq
  Min_BTrq : Constant  Value=Min_BTrq
  Subtract : Sum  Inputs=+-
  Subtract1 : Sum  Inputs=+-
  Scaling Coefficient m : Outport
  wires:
  Divide/1 -> Scaling Coefficient m/1
  Subtract1/1 -> Divide/2
  Subtract/1 -> Divide/1
  Min_BTrq/1 -> Subtract/2
  MinInputBTrq/1 -> Subtract1/2
  MaxInputBTrq/1 -> Subtract1/1
  Max_BTrq/1 -> Subtract/1

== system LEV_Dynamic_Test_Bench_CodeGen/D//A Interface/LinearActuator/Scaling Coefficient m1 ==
  Divide : Product  Inputs=*/
  MaxInputBTrq : Constant  Value=MaxInputBTrq
  Max_BTrq : Constant  Value=Max_BTrq
  MinInputBTrq : Constant  Value=MinInputBTrq
  Min_BTrq : Constant  Value=Min_BTrq
  Subtract : Sum  Inputs=+-
  Subtract1 : Sum  Inputs=+-
  Scaling Coefficient m : Outport
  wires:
  Divide/1 -> Scaling Coefficient m/1
  Subtract1/1 -> Divide/2
  Subtract/1 -> Divide/1
  Min_BTrq/1 -> Subtract/2
  MinInputBTrq/1 -> Subtract1/2
  MaxInputBTrq/1 -> Subtract1/1
  Max_BTrq/1 -> Subtract/1

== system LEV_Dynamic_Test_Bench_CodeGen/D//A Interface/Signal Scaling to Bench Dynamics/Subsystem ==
  note: Max_Signal-grad1*Digital_Output-offSet1 Min_Signal-Anglog_Input_Min*grad1-offSet1
  Anglog_Output_Max : Constant  Value=Anglog_Output_Max
  Anglog_Output_Min : Constant  Value=Anglog_Output_Min
  Divide : Product  Inputs=/*
  MaxInputBTrq : Constant  Value=MaxInputBTrq
  MinInputBTrq : Constant  Value=MinInputBTrq
  Subtract : Sum  Inputs=+-
  Subtract1 : Sum  Inputs=+-
  "Gradient " : Outport
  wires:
  Divide/1 -> "Gradient "/1
  Subtract1/1 -> Divide/2
  Subtract/1 -> Divide/1
  Anglog_Output_Min/1 -> Subtract/2
  MinInputBTrq/1 -> Subtract1/2
  MaxInputBTrq/1 -> Subtract1/1
  Anglog_Output_Max/1 -> Subtract/1

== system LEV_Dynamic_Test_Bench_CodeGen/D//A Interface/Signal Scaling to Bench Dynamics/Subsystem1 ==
  "Gradient " : Inport
  Anglog_Output_Min : Constant  Value=Anglog_Output_Min
  "MinInputBTrq " : Constant  Value=MinInputBTrq
  Product : Product
  Subtract2 : Sum  Inputs=+-
  "Offset " : Outport
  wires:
  Anglog_Output_Min/1 -> Product/1
  "Gradient "/1 -> Product/2
  Product/1 -> Subtract2/2
  Subtract2/1 -> "Offset "/1
  "MinInputBTrq "/1 -> Subtract2/1

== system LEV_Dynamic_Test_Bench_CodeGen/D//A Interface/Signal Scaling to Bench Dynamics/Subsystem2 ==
  note: Max_Signal-grad1*Digital_Output-offSet1 Min_Signal-Anglog_Input_Min*grad1-offSet1
  Anglog_Output_Max : Constant  Value=Anglog_Output_Max
  Anglog_Output_Min : Constant  Value=Anglog_Output_Min
  Divide : Product  Inputs=/*
  MaxInputBTrq : Constant  Value=MaxInputBTrq
  MinInputBTrq : Constant  Value=MinInputBTrq
  Subtract : Sum  Inputs=+-
  Subtract1 : Sum  Inputs=+-
  "Gradient " : Outport
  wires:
  Divide/1 -> "Gradient "/1
  Subtract1/1 -> Divide/2
  Subtract/1 -> Divide/1
  Anglog_Output_Min/1 -> Subtract/2
  MinInputBTrq/1 -> Subtract1/2
  MaxInputBTrq/1 -> Subtract1/1
  Anglog_Output_Max/1 -> Subtract/1

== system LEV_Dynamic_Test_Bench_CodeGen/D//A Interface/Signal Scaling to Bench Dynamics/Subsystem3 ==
  "Gradient " : Inport
  Anglog_Output_Min : Constant  Value=Anglog_Output_Min
  "MinInputBTrq " : Constant  Value=MinInputBTrq
  Product : Product
  Subtract2 : Sum  Inputs=+-
  "Offset " : Outport
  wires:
  Anglog_Output_Min/1 -> Product/1
  "Gradient "/1 -> Product/2
  Product/1 -> Subtract2/2
  Subtract2/1 -> "Offset "/1
  "MinInputBTrq "/1 -> Subtract2/1

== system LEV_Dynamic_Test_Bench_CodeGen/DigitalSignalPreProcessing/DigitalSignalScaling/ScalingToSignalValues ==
  ShaftSpeedDigitalSignal : Inport
  Divide : Product  Inputs=/**
  Full_Scale_Reading : Constant  Value=Full_Speed_Range
  Signal Specification : SignalSpecification  Unit=rad/s
  Values : Constant  Value=2^Bits -1
  "ShaftSpeedDigitalSignal " : Outport
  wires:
  ShaftSpeedDigitalSignal/1 -> Divide/2
  Values/1 -> Divide/1
  Divide/1 -> Signal Specification/1  "ShaftSpeedDigitalSignal"
  Full_Scale_Reading/1 -> Divide/3
  Signal Specification/1 -> "ShaftSpeedDigitalSignal "/1
